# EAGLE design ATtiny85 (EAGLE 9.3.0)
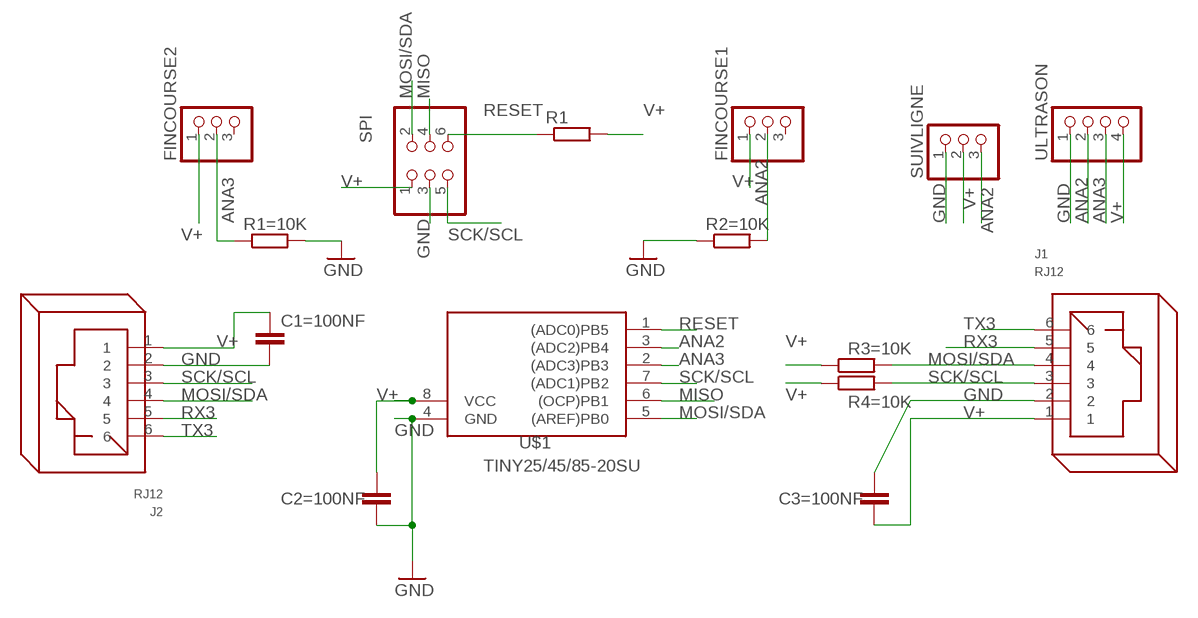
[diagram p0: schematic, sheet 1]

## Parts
C1=100NF  C-EUC1206  [C1206]
C2=100NF  C-EUC1206  [C1206]
C3=100NF  C-EUC1206  [C1206]
FINCOURSE1  PINHD-1X3  [1X03]
FINCOURSE2  PINHD-1X3  [1X03]
J1  RJ12  [RJ12]
J2  RJ12  [RJ12]
R1  R-EU_R1206  [R1206]
R1=10K  R-EU_R1206  [R1206]
R2=10K  R-EU_R1206  [R1206]
R3=10K  R-EU_R1206  [R1206]
R4=10K  R-EU_R1206  [R1206]
SPI  PINHD-2X3  [2X03]
SUIVLIGNE  PINHD-1X3  [1X03]
U$1  TINY25/45/85-20SU  [SOIC8]
ULTRASON  PINHD-1X4  [1X04]

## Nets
ANA2: FINCOURSE1.2 R2=10K.2 SUIVLIGNE.3 U$1.3((ADC2)PB4) ULTRASON.2
ANA3: FINCOURSE2.2 R1=10K.1 U$1.2((ADC3)PB3) ULTRASON.3
GND: C1=100NF.2 C2=100NF.2 C3=100NF.1 J1.2 J2.2 R1=10K.2 R2=10K.1 SPI.3 SUIVLIGNE.1 U$1.4(GND) ULTRASON.1
MISO: SPI.4 U$1.6((OCP)PB1)
MOSI/SDA: J1.4 J2.4 R3=10K.2 SPI.2 U$1.5((AREF)PB0)
RESET: R1.1 SPI.6 U$1.1((ADC0)PB5)
RX3: J1.5 J2.5
SCK/SCL: J1.3 J2.3 R4=10K.2 SPI.5 U$1.7((ADC1)PB2)
TX3: J1.6 J2.6
V+: C1=100NF.1 C2=100NF.1 C3=100NF.2 FINCOURSE1.1 FINCOURSE2.1 J1.1 J2.1 R1.2 R3=10K.1 R4=10K.1 SPI.1 SUIVLIGNE.2 U$1.8(VCC) ULTRASON.4
Unconnected: FINCOURSE1.3 FINCOURSE2.3

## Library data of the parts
C1=100NF C2=100NF C3=100NF = rcl:C-EU: CAPACITOR, European symbol; SPICEPREFIX: C
FINCOURSE1 FINCOURSE2 SUIVLIGNE = pinhead:PINHD-1X3: PIN HEADER
J1 J2 = con-rj:RJ12: RJ12, RJ14 and RJ25 RJ12, RJ14 and RJ25 jacks side mounted http://www.tycoelectronics.com
R1 R1=10K R2=10K R3=10K R4=10K = rcl:R-EU_: RESISTOR, European symbol; SPICEPREFIX: R
SPI = pinhead:PINHD-2X3: PIN HEADER
U$1 = avr-7:TINY25/45/85
ULTRASON = pinhead:PINHD-1X4: PIN HEADER

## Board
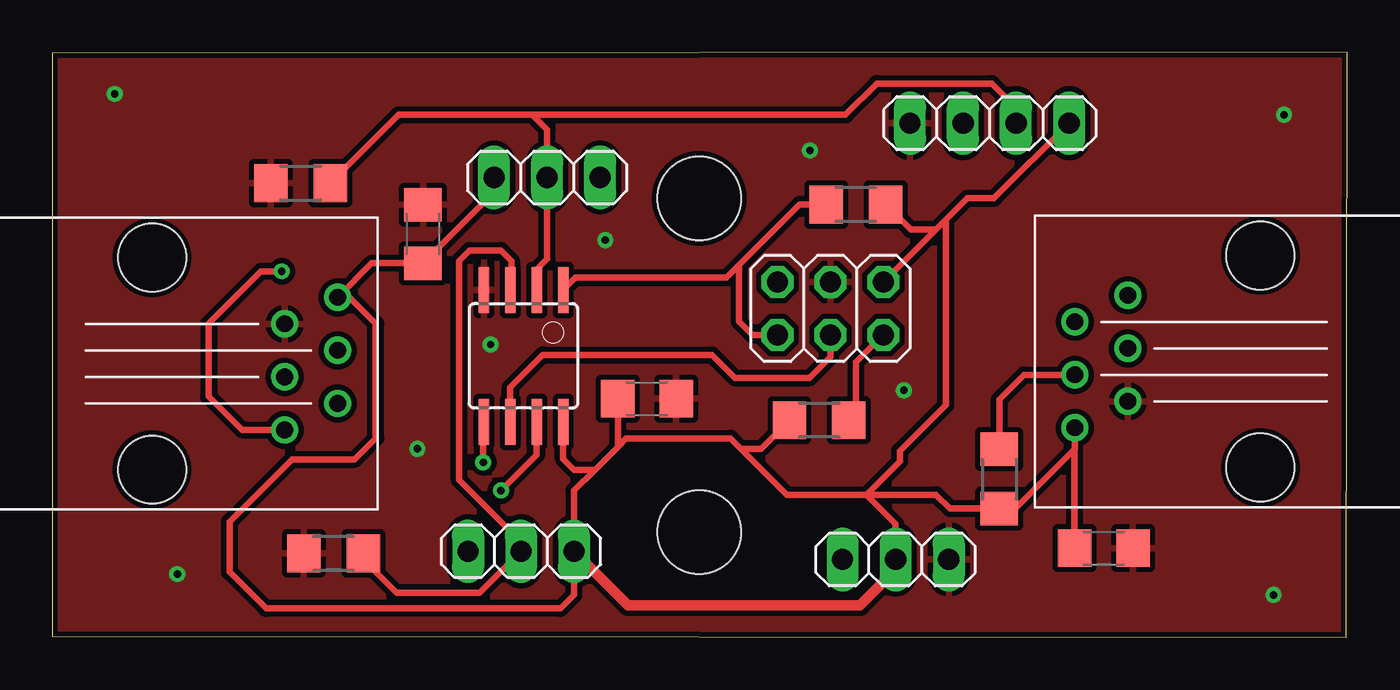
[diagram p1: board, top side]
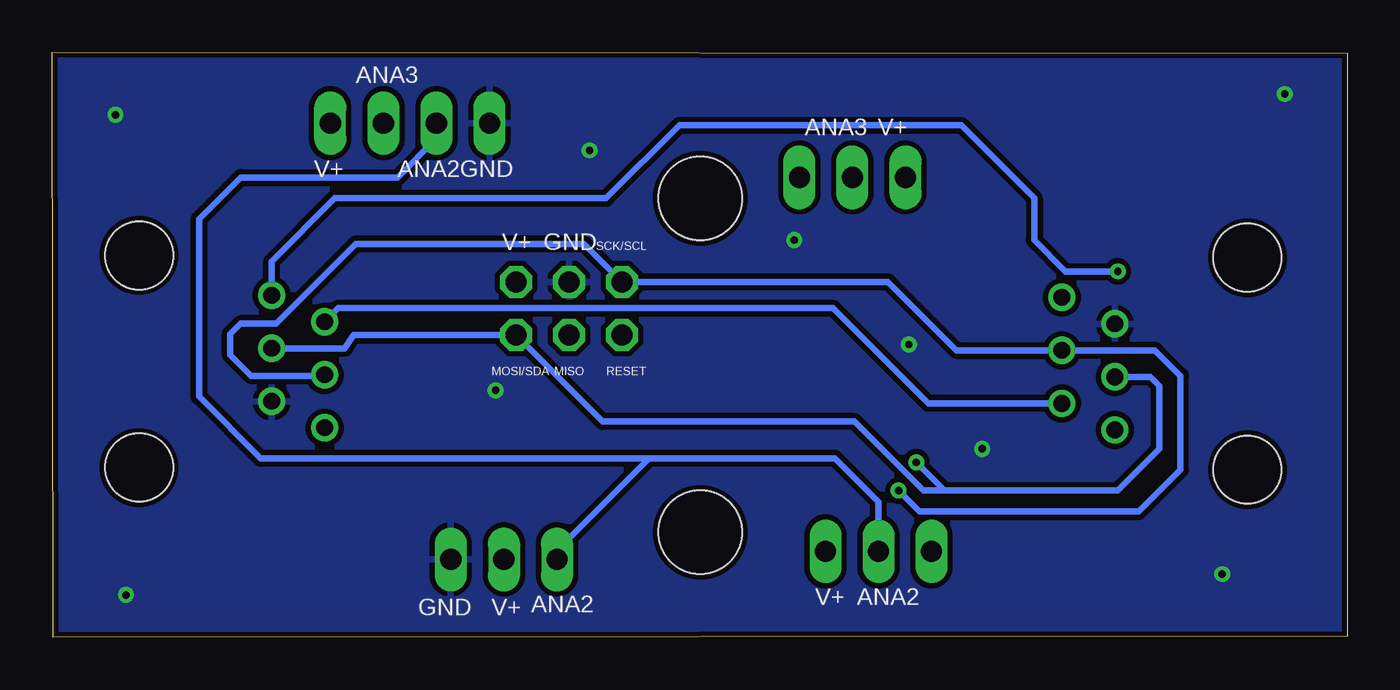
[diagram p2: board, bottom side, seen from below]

Size 62.02 x 28.04 mm. Coordinates in mm from the lower left corner, seen from the top.
Outline: 0,0.05 61.97,0 62.02,28.04 0,27.99 0,0.05
Copper layers (1*16): Top 0.035mm / dielectric 1.5mm / Bottom 0.035mm
Design rules "default *": minimum track width 6mil, minimum drill 0.35mm, track to track 8mil, track to pad 8mil, pad to pad 8mil, via to via 8mil, smd to smd 8mil, copper to edge 0.2mm, drill to drill 6mil, minimum pad ring 10mil, minimum via ring 8mil, stop-mask expansion 4mil, vias tented up to drill 0mil, thermal gap 10mil
Holes 4 mm at 30.99,5.04 30.99,21.04

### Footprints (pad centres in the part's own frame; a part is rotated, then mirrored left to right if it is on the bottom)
C1206 = smd 1.6 x 1.8: 1 -1.4,0; 2 1.4,0
1X03 = drill 1.016 long: 1 -2.54,0; 2 0,0; 3 2.54,0
RJ12 = drill 0.8: 1 -8.89,-3.175; 2 -6.35,-1.905; 3 -8.89,-0.635; 4 -6.35,0.635; 5 -8.89,1.905; 6 -6.35,3.175 | hole 3.25: 0,-5.08; 0,5.08
R1206 = smd 1.6 x 1.803: 1 -1.422,0; 2 1.422,0
2X03 = drill 1.016 octagon: 1 -2.54,-1.27; 2 -2.54,1.27; 3 0,-1.27; 4 0,1.27; 5 2.54,-1.27; 6 2.54,1.27
SOIC8 = smd 0.5 x 2.2: 1 -1.905,-3.154; 2 -0.645,-3.154; 3 0.625,-3.154; 4 1.895,-3.154; 5 1.905,3.154; 6 0.635,3.154; 7 -0.635,3.154; 8 -1.905,3.154
1X04 = drill 1.016 long: 1 -3.81,0; 2 -1.27,0; 3 1.27,0; 4 3.81,0

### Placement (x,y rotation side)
C1=100NF  50.36,4.28 0 top
C2=100NF  28.48,11.44 0 top
C3=100NF  17.75,19.33 270 top
FINCOURSE1  22.45,4.13 180 top
FINCOURSE2  23.7,22.04 0 top
J1  4.78,13.12 180 top
J2  57.86,13.22 0 top
R1  38.49,20.74 0 top
R1=10K  11.89,21.77 180 top
R2=10K  13.47,4.03 0 top
R3=10K  36.73,10.41 0 top
R4=10K  45.35,7.6 90 top
SPI  37.27,15.76 180 top
SUIVLIGNE  40.39,3.74 180 top
U$1  22.57,13.49 180 top
ULTRASON  44.89,24.64 0 top

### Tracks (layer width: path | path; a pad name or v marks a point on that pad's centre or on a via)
ANA2
  Top 0.305: U$1.3 21.99,16.69 21.99,18.04 21.49,18.54 19.99,18.54 19.49,18.04 19.49,7.54 22.45,4.58 FINCOURSE1.2 20.46,2.14 16.49,2.14 14.89,3.74 R2=10K.2
  Bottom 0.305: FINCOURSE1.2 22.45,6.5 24.54,8.59 33.43,8.59 | 33.43,8.59 37.85,4.17 SUIVLIGNE.3 | ULTRASON.2 43.62,23.91 45.49,22.04 52.99,22.04 54.99,20.04 54.99,11.54 52.04,8.59 33.43,8.59
ANA3
  Top 0.305: R1=10K.1 16.58,25.04 22.99,25.04 | 22.99,25.04 23.7,24.33 FINCOURSE2.2 23.7,18.13 23.21,17.64 U$1.2 | 22.99,25.04 37.99,25.04 39.49,26.54 44.99,26.54 46.16,25.37 ULTRASON.3
GND  (via drill 0.35)
  other vias: 5.99,3.04 17.49,9.04 20.99,14.04 36.29,23.34 58.99,25.04 58.49,2.04 2.99,26.04 26.49,19.04 40.79,11.84
  pour Bottom (isolate 0.254): 0.29,27.84 0.29,-0.16 61.99,-0.16 61.99,27.84
  pour Top (isolate 0.254): 0.29,28.04 0.29,-0.06 61.99,-0.06 61.99,28.04
MISO
  Top 0.305: U$1.6 21.93,11.98 23.49,13.54 31.59,13.54 32.69,12.44 36.27,12.44 37.27,13.44 SPI.4
MOSI/SDA  (via drill 0.35)
  Top 0.152: 20.74,10.19 U$1.5
  Top 0.305: v20.64,8.39 20.64,10.09 20.74,10.19 | R3=10K.2 38.49,10.75 38.49,13.19 39.79,14.49 SPI.2
  Bottom 0.305: J2.4 48.01,13.85 47.59,14.48 SPI.2 35.66,10.34 23.59,10.34 20.29,7.04 19.29,7.04 | v20.64,8.39 19.29,7.04 | 19.29,7.04 10.99,7.04 8.99,9.04 8.99,12.04 9.44,12.48 J1.4
RESET
  Top 0.305: U$1.1 25.07,17.24 32.29,17.24 32.89,17.84 | 32.89,17.84 32.89,15.14 33.54,14.49 SPI.6 | 32.89,17.84 35.79,20.74 R1.1
RX3
  Bottom 0.305: J1.5 20.07,11.21 24.63,15.77 48.32,15.77 J2.5
SCK/SCL  (via drill 0.35)
  Top 0.305: R4=10K.2 45.35,11.4 46.54,12.59 J2.3 | U$1.7 23.21,8.76 v21.49,7.04
  Bottom 0.305: J2.3 49.02,12.54 52.49,12.54 53.49,13.54 53.49,14.54 52.99,15.04 51.29,15.04 47.49,18.84 36.54,18.84 SPI.5 21.99,17.03 18.72,13.76 J1.3 9.21,13.76 7.99,12.54 7.99,8.04 9.99,6.04 20.49,6.04 v21.49,7.04
TX3  (via drill 0.35)
  Top 0.305: v10.99,17.54 9.99,17.54 7.49,15.04 7.49,11.54 9.09,9.95 J1.6
  Bottom 0.305: J2.6 51.51,18.02 48.49,21.04 35.49,21.04 31.99,24.54 18.49,24.54 14.99,21.04 14.99,19.04 13.49,17.54 v10.99,17.54
V+
  Top 0.305: 48.96,9.01 46.13,6.18 R4=10K.1 42.99,6.18 42.33,6.84 38.99,6.84 | 48.96,9.01 C1=100NF.1 | 42.79,20.01 42.79,11.14 40.59,8.94 40.59,8.44 38.99,6.84 | C2=100NF.1 27.09,9.14 | 25.99,8.04 24.99,8.04 24.48,8.55 U$1.8 | 25.99,8.04 27.09,9.14 | 25.99,8.04 24.99,7.04 FINCOURSE1.1 24.99,2.04 24.34,1.39 10.24,1.39 8.49,3.14 8.49,5.54 11.49,8.54 14.49,8.54 15.49,9.54 15.49,15.04 14.23,16.3 J1.1 15.3,17.93 C3=100NF.2 21.16,21.34 FINCOURSE2.1 | ULTRASON.4 45.1,21.04 43.82,21.04 42.79,20.01 | 32.99,9.04 35.19,6.84 38.99,6.84 | 48.96,9.01 48.97,9.02 J2.1 | R3=10K.1 33.94,9.04 32.99,9.04 | 38.99,6.84 40.39,5.44 SUIVLIGNE.2 | 42.32,19.54 42.79,20.01 | 42.32,19.54 41.11,19.54 R1.2 | SPI.1 42.32,19.54 | 27.09,9.14 27.49,9.54 32.49,9.54 32.99,9.04
  Top 0.508: FINCOURSE1.1 27.58,1.54 38.69,1.54 40.39,3.24 SUIVLIGNE.2

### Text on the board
bNames: ANA3 | V+ | ANA3 | GND | ANA2 | V+ | SCK/SCL | GND | V+ | RESET | MISO | MOSI/SDA | ANA2 | V+ | ANA2 | V+ | GND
